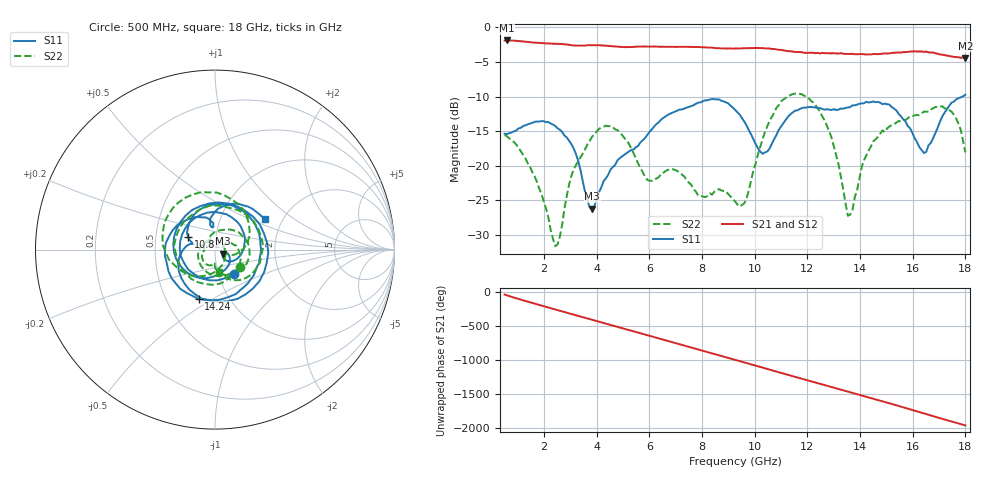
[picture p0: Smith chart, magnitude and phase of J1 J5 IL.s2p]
!Agilent Technologies,N5230A,MY45001360,A.07.50.67
!Agilent N5230A: A.07.50.67
!Date: Tuesday, April 16, 2024 16:30:02
!Correction: S11(Full 2 Port(1,2))
!S21(Full 2 Port(1,2))
!S12(Full 2 Port(1,2))
!S22(Full 2 Port(1,2))
!S2P File: Measurements: S11, S21, S12, S22:
# Hz S  dB  R 50
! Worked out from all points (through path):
!   201 points, 500 MHz to 18 GHz, reference 50 ohm
!   highest |S21| = -1.88 dB at 587.5 MHz (marker M1); lowest = -4.4 dB at 18 GHz (marker M2)
!   group delay of S21, straight-line fit = 301 ps
!   lowest |S11| = -26.2 dB at 3.825 GHz (marker M3), VSWR 1.10, Z = 54.5 - j2.39 ohm
!   |S11| at or under -10 dB: start of sweep to 17.89 GHz
!   |S22| runs from -31.6 to -9.6 dB; largest |S21 - S12| = 0.008
!   S11 on the Smith chart (normalised r, x): 500 MHz: 1.19, -0.33; 10.82 GHz: 0.73, +0.11; 14.24 GHz: 0.72, -0.43; 18 GHz: 1.63, +0.62
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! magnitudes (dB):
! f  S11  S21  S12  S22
! 500 MHz  -15.4  -1.9  -1.9  -15.6
! 587.5 MHz  -15.4  -1.9  -1.9  -15.7
! 1.637 GHz  -13.6  -2.2  -2.2  -21.5
! 2.425 GHz  -14.3  -2.4  -2.4  -31.6
! 3.038 GHz  -16.9  -2.6  -2.6  -21.5
! 3.475 GHz  -22.4  -2.6  -2.6  -18.2
! 3.825 GHz  -26.2  -2.6  -2.6  -15.8
! 4.612 GHz  -20.2  -2.7  -2.7  -14.4
! 5.925 GHz  -15.5  -2.8  -2.7  -22.1
! 6.362 GHz  -13.7  -2.8  -2.8  -21.6
! 9.25 GHz  -11.9  -3.0  -3.0  -25.1
! 9.688 GHz  -14.2  -3.0  -3.0  -24.8
! 10.3 GHz  -18.3  -3.0  -3.0  -16.1
! 10.82 GHz  -15.5  -3.2  -3.2  -11.6
! 12.22 GHz  -11.5  -3.7  -3.6  -10.9
! 12.93 GHz  -11.9  -3.7  -3.7  -16.1
! 13.54 GHz  -11.6  -3.8  -3.8  -27.2
! 14.24 GHz  -10.7  -3.9  -3.9  -18.5
! 15.11 GHz  -11.2  -3.7  -3.7  -14.3
! 16.43 GHz  -18.2  -3.5  -3.5  -12.2
! 17.48 GHz  -10.9  -4.2  -4.1  -12.2
! 18 GHz  -9.7  -4.4  -4.4  -18.1
